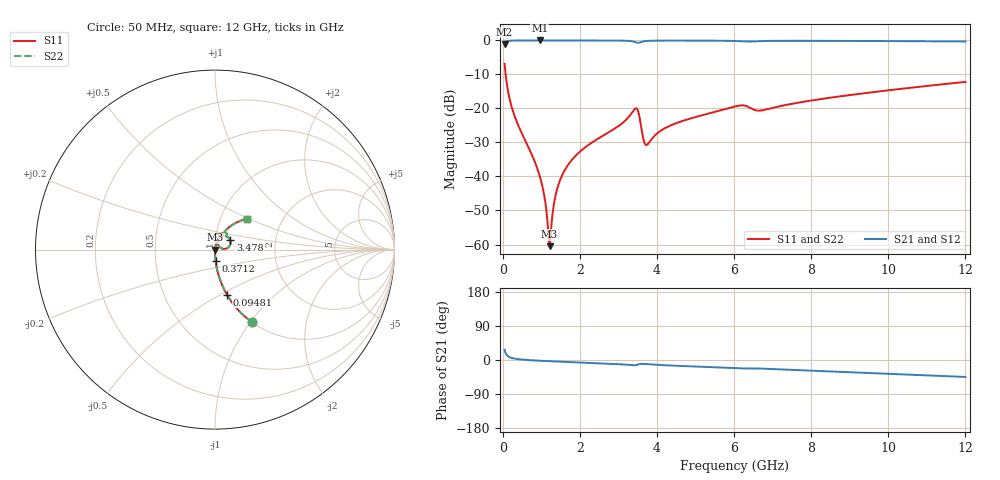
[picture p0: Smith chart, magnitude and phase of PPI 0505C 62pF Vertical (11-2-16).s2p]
# GHz S MA R 50
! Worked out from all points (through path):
!   1601 points, 50 MHz to 12 GHz, reference 50 ohm
!   highest |S21| = -0.01 dB at 961.2 MHz (marker M1); lowest = -1.0 dB at 50 MHz (marker M2)
!   group delay of S21, straight-line fit = 10.8 ps
!   lowest |S11| = -60.5 dB at 1.215 GHz (marker M3), VSWR 1.00, Z = 50.1 - j0.00925 ohm
!   |S11| at or under -10 dB: 76.56 MHz to end of sweep
!   |S22| runs from -60.5 to -6.8 dB; largest |S21 - S12| = 0
!   S11 on the Smith chart (normalised r, x): 50 MHz: 1.00, -1.02; 94.81 MHz: 1.00, -0.54; 371.2 MHz: 1.00, -0.13; 3.478 GHz: 1.18, +0.12; 12 GHz: 1.33, +0.48
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0.05  0.4551 -63.0  0.8902 26.9  0.8902 26.9  0.4551 -63.0
0.0948125  0.2592 -75.2  0.9655 14.8  0.9655 14.8  0.2592 -75.2
0.199375  0.124 -83.2  0.9918 6.6  0.9918 6.6  0.124 -83.2
0.3711563  0.0625 -86.9  0.9975 2.6  0.9975 2.6  0.0625 -86.9
0.9611875  0.01013 -87.1  0.999 -1.9  0.999 -1.9  0.01013 -87.1
1.073219  0.005421 -83.0  0.999 -2.5  0.999 -2.5  0.005421 -83.0
1.177781  0.00166 -58.9  0.999 -3.0  0.999 -3.0  0.00166 -58.9
1.215125  0.0009452 -5.6  0.999 -3.2  0.999 -3.2  0.0009452 -5.6
1.252469  0.00158 49.3  0.999 -3.3  0.999 -3.3  0.00158 49.3
1.3645  0.005057 74.8  0.9989 -3.9  0.9989 -3.9  0.005057 74.8
1.491469  0.008938 78.9  0.9988 -4.4  0.9988 -4.4  0.008938 78.9
1.715531  0.01536 80.4  0.9986 -5.4  0.9986 -5.4  0.01536 80.4
2.044156  0.02424 80.2  0.9983 -6.7  0.9983 -6.7  0.02424 80.2
3.478156  0.09945 31.5  0.9265 -13.1  0.9265 -13.1  0.09945 31.5
3.709687  0.02921 33.0  0.9785 -10.8  0.9785 -10.8  0.02921 33.0
4.038312  0.04445 69.2  0.9928 -13.0  0.9928 -13.0  0.04445 69.2
4.620875  0.06427 71.3  0.9942 -15.7  0.9942 -15.7  0.06427 71.3
6.025  0.107 61.5  0.9813 -21.7  0.9813 -21.7  0.107 61.5
6.674781  0.09305 55.7  0.9764 -22.5  0.9764 -22.5  0.09305 55.7
8.019156  0.1313 59.9  0.9865 -28.2  0.9865 -28.2  0.1313 59.9
10.01331  0.1852 52.5  0.9784 -36.3  0.9784 -36.3  0.1852 52.5
12  0.2457 44.3  0.9647 -44.8  0.9647 -44.8  0.2457 44.3
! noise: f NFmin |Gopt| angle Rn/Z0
0.05  0.0003693  0.8579  0.4763  0.0005557
1.372  0.003757  0.6576  3.56  0.002092
2.701  0.007534  0.663  6.837  0.004266
4.031  0.01576  0.7478  10.39  0.01247
5.36  0.01474  0.6603  13.49  0.008188
6.682  0.03547  0.8087  17.17  0.03776
8.012  0.01913  0.6206  19.77  0.009146
9.341  0.01913  0.5729  22.44  0.007828
10.67  0.02059  0.5545  25.14  0.007913
12  0.02251  0.5469  27.8  0.008381
